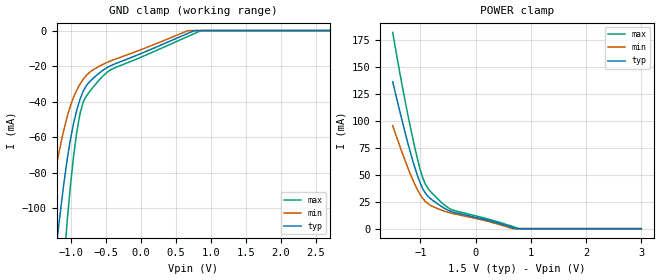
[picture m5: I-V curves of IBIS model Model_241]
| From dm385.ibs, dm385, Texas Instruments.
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| Model based on original model for BCSHTLTCSCDVPBFZ_SSDHV
|   Sub model VREF_FULLTERM_7MA_10PER_1P5
[model]   Model_241
|[Description]  [1.5V-INPUT-FULLTERM:7MA-X, IND, 10%]
|   FULLTERM, 1.14 * RExt = 0.875 * Iout (I[2:0] = "010"), 7mA
|   nominal with Rext = 50R,Industrial temperature range (-40C to
|   125C, 25C nominal),10% power supply tolerance
|[Input Load]   FULLTERM:7MA
|[Output Drive]
|Voltage   1.5V
|Mode   INPUT
Model_type   Input
Polarity   Non-Inverting
Vinl =  0.65
Vinh =  0.85
C_comp   1.865048p   1.676829p   1.989968p
[Model Spec]
Vinl   0.65   0.575   0.725
Vinh   0.85   0.775   0.925
[Temperature Range]   25   125   -40
[Voltage Range]   1.5   1.35   1.65
[POWER_clamp]
-1.5V     136.3mA    95.48mA    182mA
-1.364V   107.1mA    75.48mA    142.4mA
-1.227V   79.59mA    56.69mA    106mA
-1.091V   55.26mA    40.15mA    73.22mA
-1V       42.05mA    31.31mA    54.45mA
-954.5mV  36.86mA    27.88mA    46.87mA
-863.6mV  30.07mA    23.23mA    37.4mA
-545.5mV  18.4mA     15.92mA    21.21mA
-363.6mV  14.75mA    13.49mA    16.47mA
681.8mV   836.4uA    0A         1.806mA
772.7mV   0A         0A         257.8uA
3V        0A         0A         0A
[GND_clamp]
-1.5V     -235.2mA   -143.5mA   -381.7mA
-1.364V   -181.6mA   -111.4mA   -293.3mA
-1.182V   -114.4mA   -71.88mA   -180mA
-1.091V   -84.63mA   -55.06mA   -128.5mA
-1.045V   -71.81mA   -47.99mA   -106mA
-954.5mV  -51.77mA   -37.17mA   -69.96mA
-863.6mV  -38.5mA    -30mA      -46.4mA
-818.2mV  -33.95mA   -27.31mA   -40.02mA
-681.8mV  -27.01mA   -22.16mA   -32.01mA
-409.1mV  -19.41mA   -16.76mA   -21.67mA
863.6mV   0A         0A         0A
3V        0A         0A         0A
